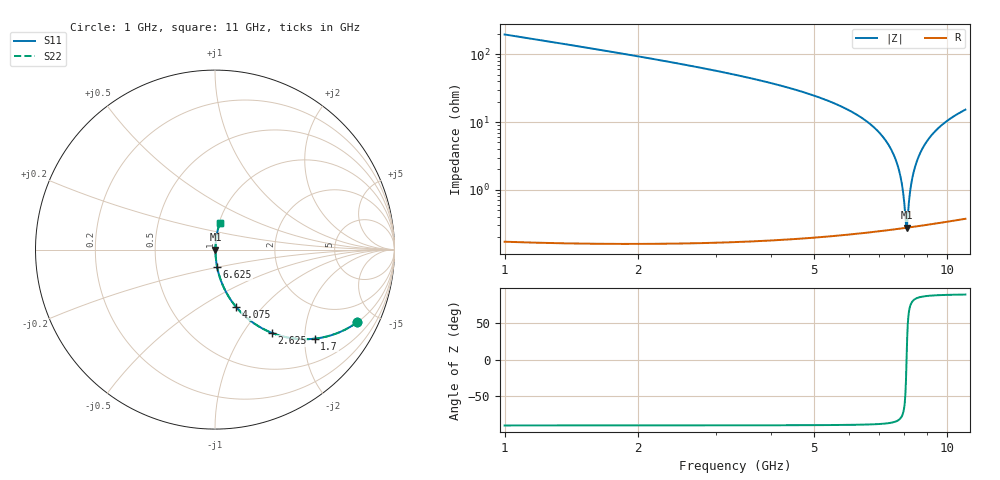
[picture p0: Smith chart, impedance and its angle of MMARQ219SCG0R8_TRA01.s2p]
! MMARQ219SCG0R8_TRA01  S-PARAMETER MODEL  ( General Type )
! Model Generated by TAIYO YUDEN Corporation (http://www.ty-top.com)
! Version 1.0
! TAIYO YUDEN Control No. 180601
! Copyright(c) 2018 TAIYO YUDEN CO.,LTD. All Rights Reserved.
! Product Description (link to TY-COMPAS)
! https://ds.yuden.co.jp/TYCOMPAS/or/detail?pn=MMARQ219SCG0R8BTRA01&u=M
! Products Name : Multilayer Ceramic Capacitors
! Characteristics :
!  Capacitance : 0.8 pF , Rated Voltage : 250V , TCC : CG / C0G
!  Case Size : 2.0 x 1.25 / 0.079 x 0.049 [mm/inch] , Thickness : 0.85 / 0.033 [mm/inch]
!  (Conditions: Temperature = 25 degC , DC Bias Current/Voltage = 0A / 0V)
! External Node Assignments :
!  1  o---| |---o  2
! GND o---------o GND
! Frequency Range : 1000MHz  -  11000MHz  [ 401 STEP ]
# MHz S RI R 50
! Freq[MHz].  S11 Real  S11 Imag  S21 Real  S21 Imag  S12 Real  S12 Imag  S22 Real  S22 Imag
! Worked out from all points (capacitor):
!   401 points, 1 GHz to 11 GHz, reference 50 ohm
!   read as one part in series: C = 800 fF near 1.05 GHz
!   lowest |Z| = 276 mohm at 8.1 GHz (marker M1)
!   series resonance near 8.099 GHz, so ESL is about 480 pH
!   S11 on the Smith chart (normalised r, x): 1 GHz: 1.00, -3.92; 1.7 GHz: 1.00, -2.24; 2.625 GHz: 1.00, -1.36; 4.075 GHz: 1.00, -0.73; 6.625 GHz: 1.00, -0.20; 11 GHz: 1.01, +0.30
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1000  0.793 -0.4047  0.207 0.4047  0.207 0.4047  0.793 -0.4047
1700  0.5556 -0.4962  0.4444 0.4962  0.4444 0.4962  0.5556 -0.4962
2625  0.3154 -0.4635  0.6846 0.4635  0.6846 0.4635  0.3154 -0.4635
2675  0.3054 -0.4593  0.6946 0.4593  0.6946 0.4593  0.3054 -0.4593
4075  0.1184 -0.3207  0.8816 0.3207  0.8816 0.3207  0.1184 -0.3207
4350  0.097 -0.2931  0.903 0.2931  0.903 0.2931  0.097 -0.2931
6000  0.0239 -0.1456  0.9761 0.1456  0.9761 0.1456  0.0239 -0.1456
6625  0.012 -0.0978  0.988 0.0978  0.988 0.0978  0.012 -0.0978
7250  0.00544 -0.054  0.9946 0.054  0.9946 0.054  0.00544 -0.054
7675  0.00332 -0.0262  0.9967 0.0262  0.9967 0.0262  0.00332 -0.0262
7900  0.00284 -0.0121  0.9972 0.0121  0.9972 0.0121  0.00284 -0.0121
7975  0.00278 -0.00753  0.9972 0.00753  0.9972 0.00753  0.00278 -0.00753
8050  0.00275 -0.00296  0.9972 0.00296  0.9972 0.00296  0.00275 -0.00296
8100  0.00276 6.21e-05  0.9972 -6.21e-05  0.9972 -6.21e-05  0.00276 6.21e-05
8150  0.00278 0.00306  0.9972 -0.00306  0.9972 -0.00306  0.00278 0.00306
8225  0.00285 0.00753  0.9971 -0.00753  0.9971 -0.00753  0.00285 0.00753
8300  0.00296 0.012  0.997 -0.012  0.997 -0.012  0.00296 0.012
8500  0.00344 0.0236  0.9966 -0.0236  0.9966 -0.0236  0.00344 0.0236
8850  0.00487 0.0432  0.9951 -0.0432  0.9951 -0.0432  0.00487 0.0432
9350  0.00808 0.0699  0.9919 -0.0699  0.9919 -0.0699  0.00808 0.0699
10075  0.0148 0.1059  0.9852 -0.1059  0.9852 -0.1059  0.0148 0.1059
11000  0.0262 0.1478  0.9738 -0.1478  0.9738 -0.1478  0.0262 0.1478
